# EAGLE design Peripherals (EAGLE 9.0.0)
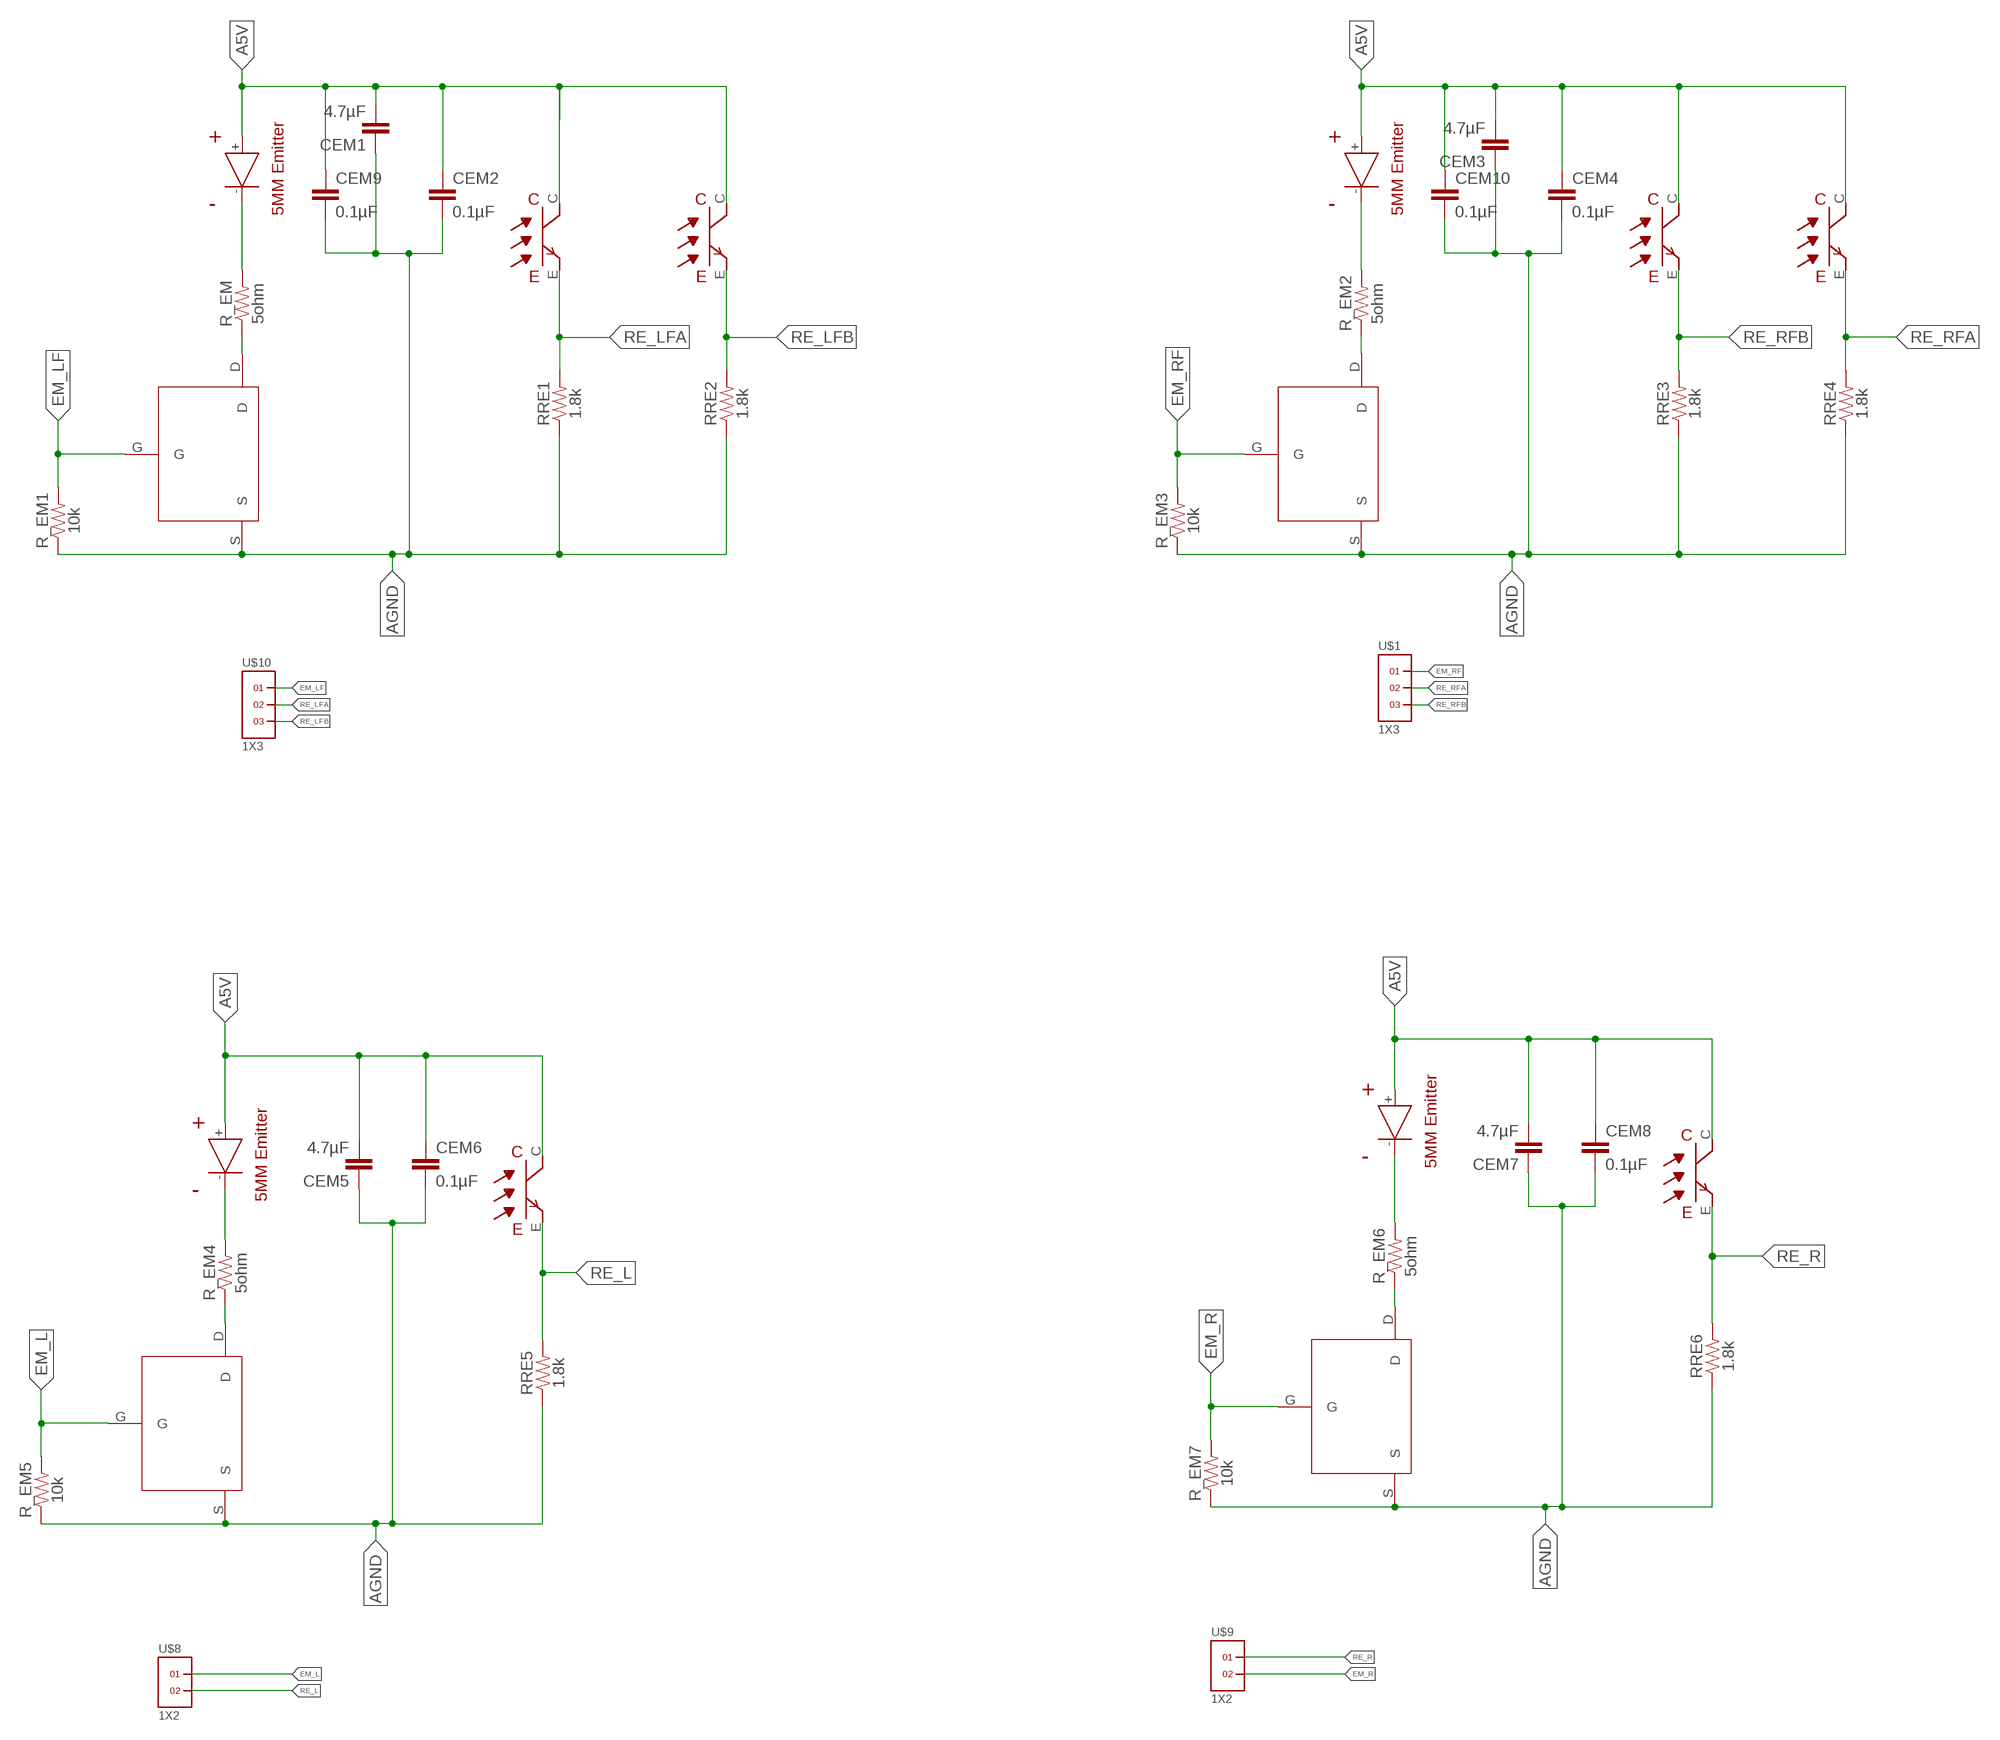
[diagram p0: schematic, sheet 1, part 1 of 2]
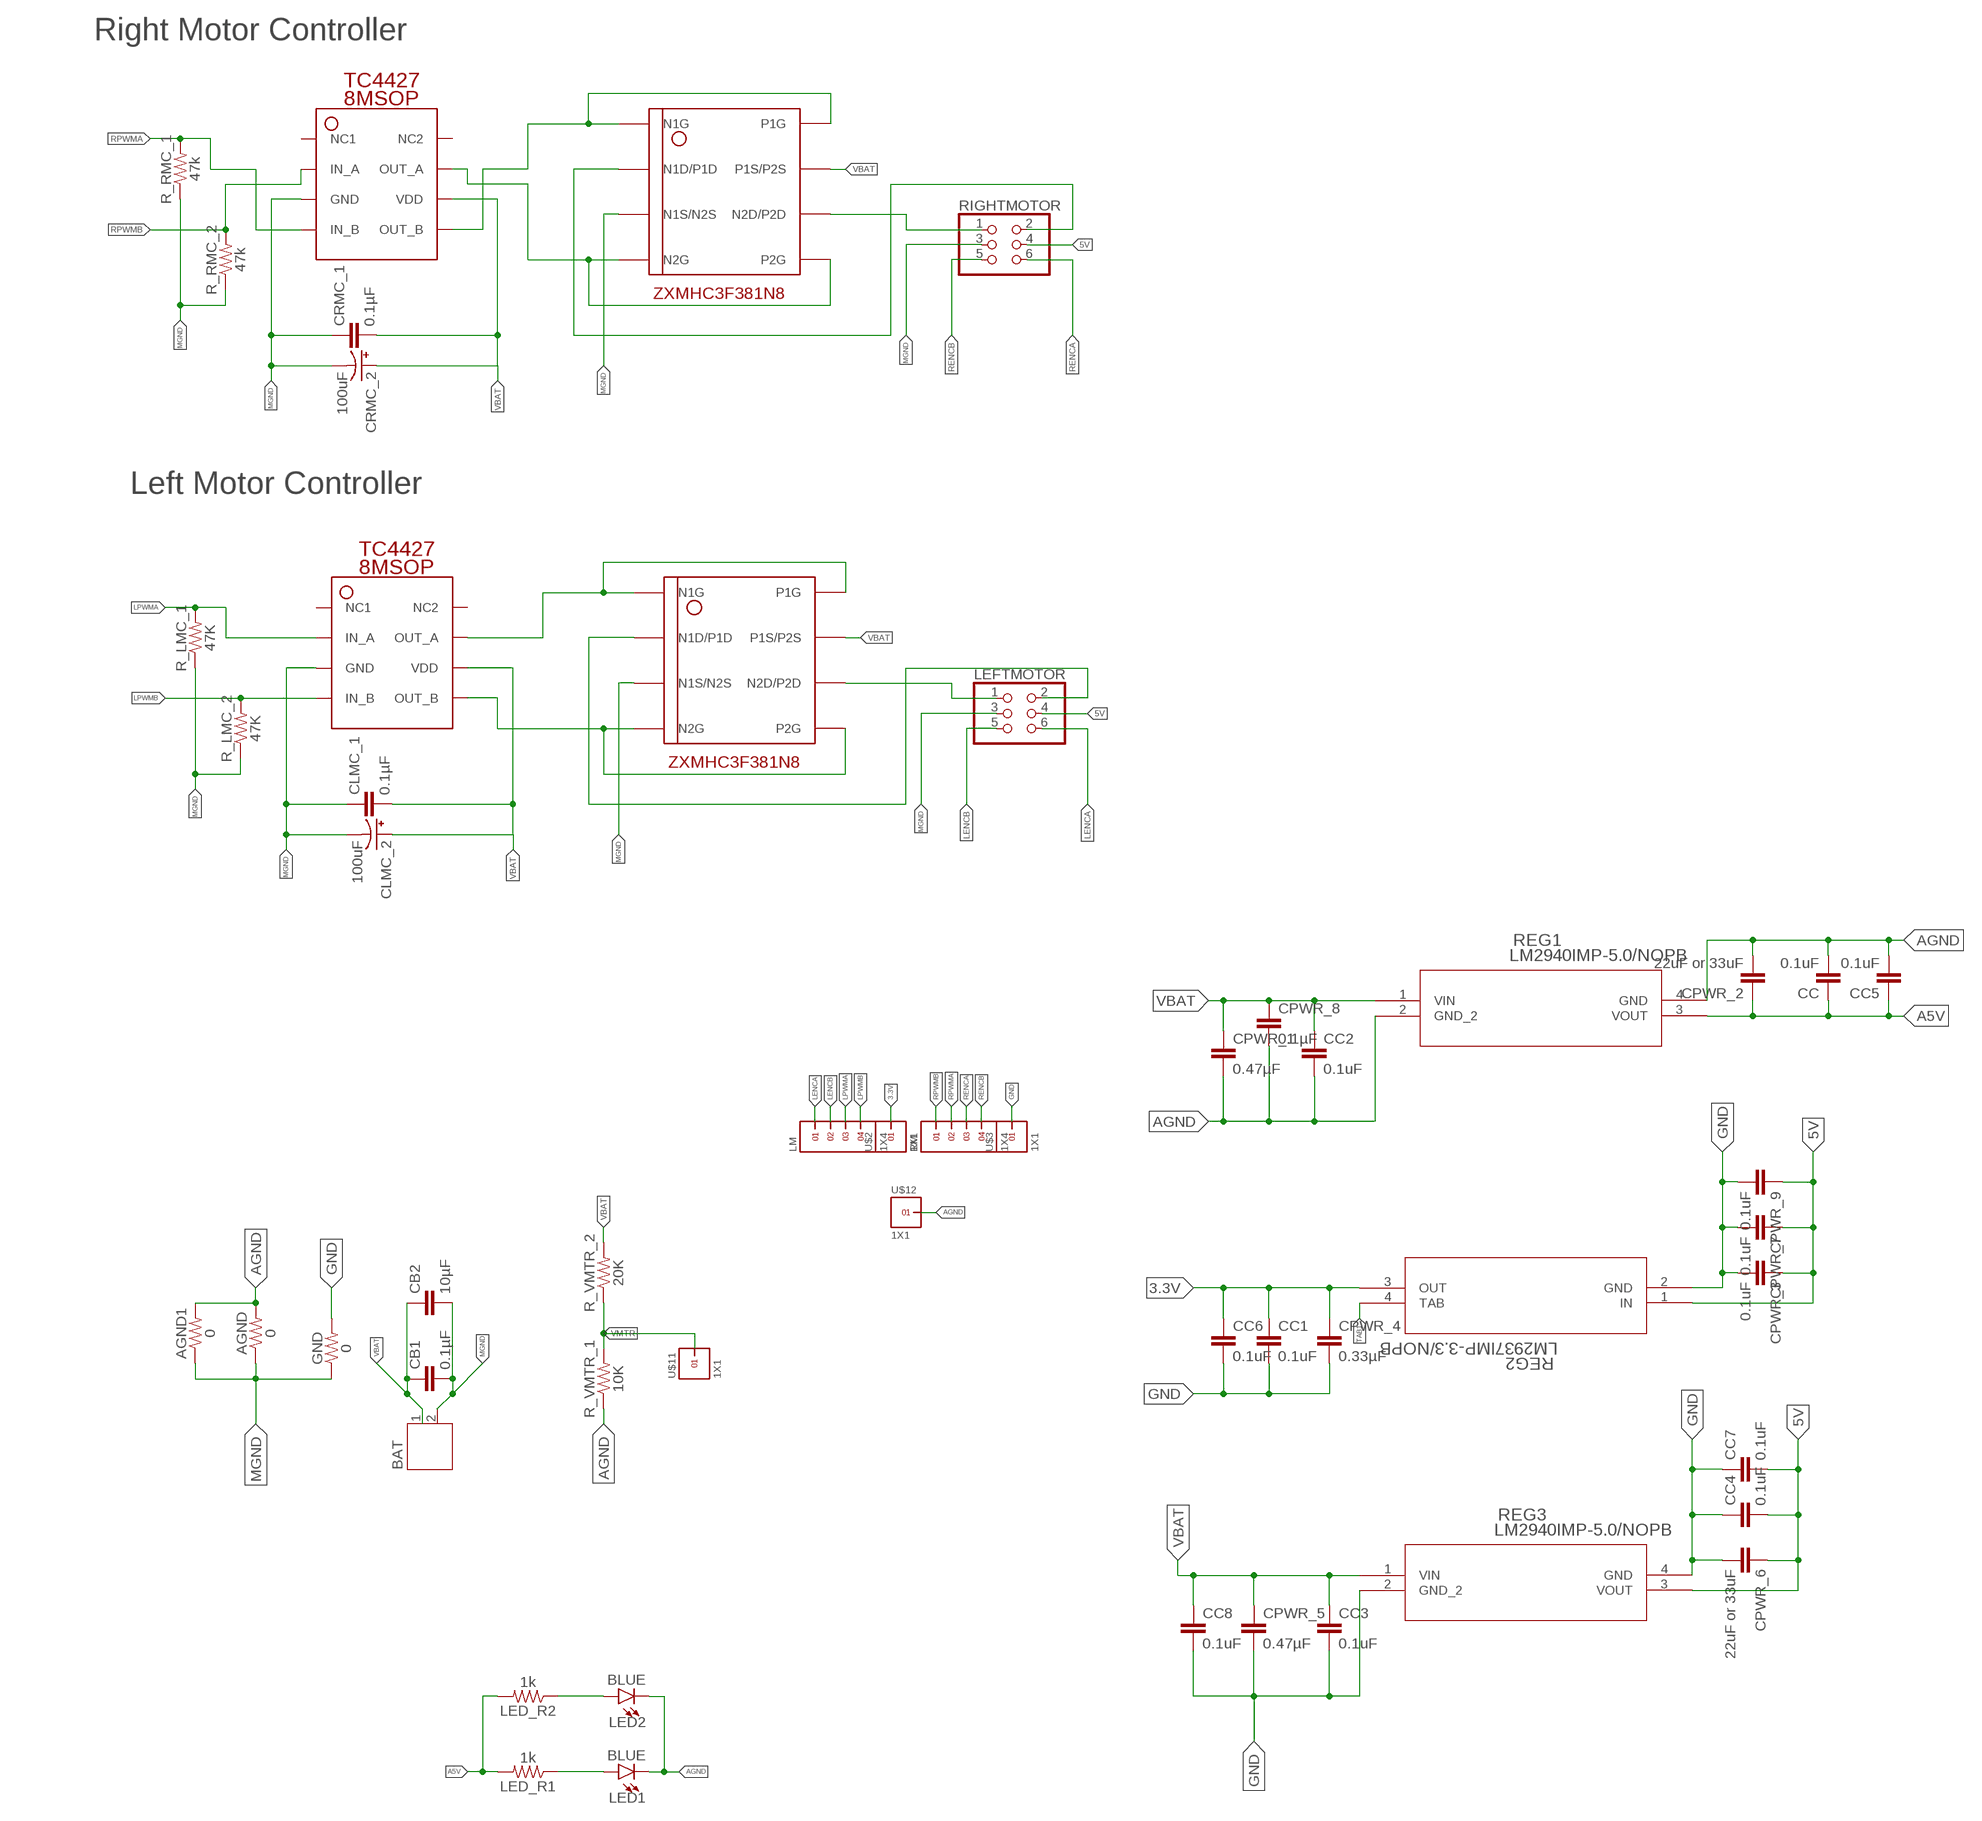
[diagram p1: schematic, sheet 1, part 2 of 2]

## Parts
AGND  0  0.75OHM-0805-1/4W-1%  [0805]
AGND1  0  0.75OHM-0805-1/4W-1%  [0805]
BAT  JST-PH2  [JST-PH2]
CB1  0.1µF  0.33UF/330NF-0805-50V-10%  [0805]
CB2  10µF  0.33UF/330NF-0805-50V-10%  [0805]
CC  0.1uF  0.33UF/330NF-0805-50V-10%  [0805]
CC1  0.1uF  0.33UF/330NF-0805-50V-10%  [0805]
CC2  0.1uF  0.33UF/330NF-0805-50V-10%  [0805]
CC3  0.1uF  0.33UF/330NF-0805-50V-10%  [0805]
CC4  0.1uF  0.33UF/330NF-0805-50V-10%  [0805]
CC5  0.1uF  0.33UF/330NF-0805-50V-10%  [0805]
CC6  0.1uF  0.33UF/330NF-0805-50V-10%  [0805]
CC7  0.1uF  0.33UF/330NF-0805-50V-10%  [0805]
CC8  0.1uF  0.33UF/330NF-0805-50V-10%  [0805]
CEM1  4.7µF  0.33UF/330NF-0805-50V-10%  [0805]
CEM2  0.1µF  0.33UF/330NF-0805-50V-10%  [0805]
CEM3  4.7µF  0.33UF/330NF-0805-50V-10%  [0805]
CEM4  0.1µF  0.33UF/330NF-0805-50V-10%  [0805]
CEM5  4.7µF  0.33UF/330NF-0805-50V-10%  [0805]
CEM6  0.1µF  0.33UF/330NF-0805-50V-10%  [0805]
CEM7  4.7µF  0.33UF/330NF-0805-50V-10%  [0805]
CEM8  0.1µF  0.33UF/330NF-0805-50V-10%  [0805]
CEM9  0.1µF  0.33UF/330NF-0805-50V-10%  [0805]
CEM10  0.1µF  0.33UF/330NF-0805-50V-10%  [0805]
CLMC_1  0.1µF  0.33UF/330NF-0805-50V-10%  [0805]
CLMC_2  100uF  100UF-POLAR-EIA7343-10V-10%(TANT)  [EIA7343]
CPWR_1  0.47µF  0.33UF/330NF-0805-50V-10%  [0805]
CPWR_2  22uF or 33uF  0.33UF/330NF-0805-50V-10%  [0805]
CPWR_3  0.1uF  0.33UF/330NF-0805-50V-10%  [0805]
CPWR_4  0.33µF  0.33UF/330NF-0805-50V-10%  [0805]
CPWR_5  0.47µF  0.33UF/330NF-0805-50V-10%  [0805]
CPWR_6  22uF or 33uF  0.33UF/330NF-0805-50V-10%  [0805]
CPWR_7  0.1uF  0.33UF/330NF-0805-50V-10%  [0805]
CPWR_8  0.1µF  0.33UF/330NF-0805-50V-10%  [0805]
CPWR_9  0.1uF  0.33UF/330NF-0805-50V-10%  [0805]
CRMC_1  0.1µF  0.33UF/330NF-0805-50V-10%  [0805]
CRMC_2  100uF  100UF-POLAR-EIA7343-10V-10%(TANT)  [EIA7343]
EM_L  EMITTER  [EMITTER]
EM_LF  EMITTER  [EMITTER]
EM_R  EMITTER  [EMITTER]
EM_RF  EMITTER  [EMITTER]
GND  0  0.75OHM-0805-1/4W-1%  [0805]
LED1  BLUE  LED-BLUE1206  [LED-1206]
LED2  BLUE  LED-BLUE1206  [LED-1206]
LED_R1  1k  0.75OHM-0805-1/4W-1%  [0805]
LED_R2  1k  0.75OHM-0805-1/4W-1%  [0805]
LEFTMOTOR  PINHD-2X3  [2X03]
LM  1X4  [1X4]
R_EM  5ohm  0.75OHM-0805-1/4W-1%  [0805]
R_EM1  10k  0.75OHM-0805-1/4W-1%  [0805]
R_EM2  5ohm  0.75OHM-0805-1/4W-1%  [0805]
R_EM3  10k  0.75OHM-0805-1/4W-1%  [0805]
R_EM4  5ohm  0.75OHM-0805-1/4W-1%  [0805]
R_EM5  10k  0.75OHM-0805-1/4W-1%  [0805]
R_EM6  5ohm  0.75OHM-0805-1/4W-1%  [0805]
R_EM7  10k  0.75OHM-0805-1/4W-1%  [0805]
R_LMC_1  47K  0.75OHM-0805-1/4W-1%  [0805]
R_LMC_2  47K  0.75OHM-0805-1/4W-1%  [0805]
R_RMC_1  47k  0.75OHM-0805-1/4W-1%  [0805]
R_RMC_2  47k  0.75OHM-0805-1/4W-1%  [0805]
R_VMTR_1  10K  0.75OHM-0805-1/4W-1%  [0805]
R_VMTR_2  20K  0.75OHM-0805-1/4W-1%  [0805]
RE_L  RECEIVER  [RECEIVER]
RE_LFA  RECEIVER  [RECEIVER]
RE_LFB  RECEIVER  [RECEIVER]
RE_R  RECEIVER  [RECEIVER]
RE_RFA  RECEIVER  [RECEIVER]
RE_RFB  RECEIVER  [RECEIVER]
REG1  LM2940IMP-5.0/NOPB  [MP04A]
REG2  LM2937IMP-3.3/NOPB  [MP04A]
REG3  LM2940IMP-5.0/NOPB  [MP04A]
RIGHTMOTOR  PINHD-2X3  [2X03]
RM  1X4  [1X4]
RRE1  1.8k  0.75OHM-0805-1/4W-1%  [0805]
RRE2  1.8k  0.75OHM-0805-1/4W-1%  [0805]
RRE3  1.8k  0.75OHM-0805-1/4W-1%  [0805]
RRE4  1.8k  0.75OHM-0805-1/4W-1%  [0805]
RRE5  1.8k  0.75OHM-0805-1/4W-1%  [0805]
RRE6  1.8k  0.75OHM-0805-1/4W-1%  [0805]
U$1  1X3  [1X3]
U$2  1X1  [1X1]
U$3  1X1  [1X1]
U$4  MCH3474  [MCH3474]
U$5  MCH3474  [MCH3474]
U$6  MCH3474  [MCH3474]
U$7  MCH3474  [MCH3474]
U$8  1X2  [1X2]
U$9  1X2  [1X2]
U$10  1X3  [1X3]
U$11  1X1  [1X1]
U$12  1X1  [1X1]
U$15  TC4427(8MSOP)  [TC4427(8MSOP)]
U$16  ZXMHC3F381N8  [ZXMHC3F381N8]
U$17  TC4427(8MSOP)  [TC4427(8MSOP)]
U$18  ZXMHC3F381N8  [ZXMHC3F381N8]

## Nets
3.3V: CC1.1 CC6.1 CPWR_4.1 REG2.3(OUT) U$2.1
5V: CC4.2 CC7.2 CPWR_3.1 CPWR_6.1 CPWR_7.1 CPWR_9.1 LEFTMOTOR.4 REG2.1(IN) REG3.3(VOUT) RIGHTMOTOR.4
A5V: CC5.1 CC.1 CEM1.2 CEM2.1 CEM3.2 CEM4.1 CEM5.2 CEM6.1 CEM7.2 CEM8.1 CEM9.1 CEM10.1 CPWR_2.1 EM_L.+ EM_LF.+ EM_R.+ EM_RF.+ LED_R1.2 LED_R2.2 RE_L.C RE_LFA.C RE_LFB.C RE_R.C RE_RFA.C RE_RFB.C REG1.3(VOUT)
AGND: AGND1.2 AGND.2 CC2.2 CC5.2 CC.2 CEM1.1 CEM2.2 CEM3.1 CEM4.2 CEM5.1 CEM6.2 CEM7.1 CEM8.2 CEM9.2 CEM10.2 CPWR_1.2 CPWR_2.2 CPWR_8.2 LED1.C LED2.C R_EM1.1 R_EM3.1 R_EM5.1 R_EM7.1 R_VMTR_1.1 REG1.2(GND_2) REG1.4(GND) RRE1.1 RRE2.1 RRE3.1 RRE4.1 RRE5.1 RRE6.1 U$4.S U$5.S U$6.S U$7.S U$12.1
EM_L: R_EM5.2 U$4.G U$8.1
EM_LF: R_EM1.2 U$5.G U$10.1
EM_R: R_EM7.2 U$7.G U$9.2
EM_RF: R_EM3.2 U$1.1 U$6.G
EMD_L: EM_L.- R_EM4.2
GND: CC1.2 CC3.2 CC4.1 CC6.2 CC7.1 CC8.2 CPWR_3.2 CPWR_4.2 CPWR_5.2 CPWR_6.2 CPWR_7.2 CPWR_9.2 GND.2 REG2.2(GND) REG3.2(GND_2) REG3.4(GND) U$3.1
L: LEFTMOTOR.2 U$16.N1D/P1D
LENCA: LEFTMOTOR.6 LM.1
LENCB: LEFTMOTOR.5 LM.2
LPWMA: LM.3 R_LMC_1.2 U$15.IN_A
LPWMB: LM.4 R_LMC_2.2 U$15.IN_B
MGND: AGND1.1 AGND.1 BAT.2 CB1.2 CB2.2 CLMC_1.1 CLMC_2.C(-) CRMC_1.1 CRMC_2.C(-) GND.1 LEFTMOTOR.3 R_LMC_1.1 R_LMC_2.1 R_RMC_1.1 R_RMC_2.1 RIGHTMOTOR.3 U$15.GND U$16.N1S/N2S U$17.GND U$18.N1S/N2S
N$1: R_EM.1 U$5.D
N$2: R_EM2.1 U$6.D
N$3: R_EM4.1 U$4.D
N$4: R_EM6.1 U$7.D
N$5: EM_LF.- R_EM.2
N$6: EM_RF.- R_EM2.2
N$7: EM_R.- R_EM6.2
N$8: LED1.A LED_R1.1
N$9: LEFTMOTOR.1 U$16.N2D/P2D
N$10: LED2.A LED_R2.1
N$36: RIGHTMOTOR.1 U$18.N2D/P2D
OUT_A: U$15.OUT_A U$16.N1G U$16.P1G
OUT_B: U$15.OUT_B U$16.N2G U$16.P2G
OUTA: U$17.OUT_B U$18.N1G U$18.P1G
OUTB: U$17.OUT_A U$18.N2G U$18.P2G
R: RIGHTMOTOR.2 U$18.N1D/P1D
RE_L: RE_L.E RRE5.2 U$8.2
RE_LFA: RE_LFA.E RRE1.2 U$10.2
RE_LFB: RE_LFB.E RRE2.2 U$10.3
RE_R: RE_R.E RRE6.2 U$9.1
RE_RFA: RE_RFB.E RRE4.2 U$1.2
RE_RFB: RE_RFA.E RRE3.2 U$1.3
RENCA: RIGHTMOTOR.6 RM.3
RENCB: RIGHTMOTOR.5 RM.4
RPWMA: R_RMC_1.2 RM.2 U$17.IN_B
RPWMB: R_RMC_2.2 RM.1 U$17.IN_A
TAB1: REG2.4(TAB)
VBAT: BAT.1 CB1.1 CB2.1 CC2.1 CC3.1 CC8.1 CLMC_1.2 CLMC_2.A(+) CPWR_1.1 CPWR_5.1 CPWR_8.1 CRMC_1.2 CRMC_2.A(+) R_VMTR_2.2 REG1.1(VIN) REG3.1(VIN) U$15.VDD U$16.P1S/P2S U$17.VDD U$18.P1S/P2S
VMTR: R_VMTR_1.2 R_VMTR_2.1 U$11.1
Unconnected: U$15.NC1 U$15.NC2 U$17.NC1 U$17.NC2

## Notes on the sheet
- Right Motor Controller
- Left Motor Controller

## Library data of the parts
AGND AGND1 GND LED_R1 LED_R2 R_EM R_EM1-R_EM7 R_LMC_1 R_LMC_2 R_RMC_1 R_RMC_2 R_VMTR_1 R_VMTR_2 RRE1-RRE6 = SparkFun-Resistors:0.75OHM: 0.75Ω resistor; PROD_ID: RES-08474; VALUE: 0.75
BAT = jst-ph:JST-PH2
CB1 CB2 CC CC1-CC8 CEM1-CEM10 CLMC_1 CPWR_1-CPWR_3 CPWR_5-CPWR_9 CRMC_1 = SparkFun-Capacitors:0.33UF/330NF: 0.33µF/330nF ceramic capacitors; PROD_ID: CAP-08469; VALUE: 0.33µF
CLMC_2 CRMC_2 = SparkFun-Capacitors:100UF-POLAR: 100µF polarized capacitors; PROD_ID: CAP-07890
CPWR_4 = SparkFun-Capacitors:0.33UF/330NF: 0.33µF/330nF ceramic capacitors; PROD_ID: CAP-08469
EM_L EM_LF EM_R EM_RF = sfh4550 & teft4300:EMITTER
LED1 LED2 = SparkFun-LED:LED-BLUE: Blue SMD LED; PROD_ID: DIO-09911
LEFTMOTOR RIGHTMOTOR = pinhead:PINHD-2X3: PIN HEADER
LM RM = headers(2mm):1X4
RE_L RE_LFA RE_LFB RE_R RE_RFA RE_RFB = sfh4550 & teft4300:RECEIVER
REG1 REG3 = LM2940IMP-5.0:LM2940IMP-5.0/NOPB; 3D_LIBRARY_NAME: National_LDO; BASE_PN: LM2940; COMP: TypeLDO; COPYRIGHT: Copyright C 2015 Accelerated Designs. All rights reserved; LIBRARY: ReferenceLM2940IMP; MANUFACTURER_PART_NUMBER: LM2940IMP5.0NOPB; PIN: Count4; SYMBOL: NameLM2940IMP50; TYPE: LM2940IMP5.0; VENDOR: National Semiconductor; VERSION: 1
REG2 = LM2937IMP-3.3:LM2937IMP-3.3/NOPB; COPYRIGHT: Copyright C 2015 Accelerated Designs. All rights reserved; MANUFACTURER_PART_NUMBER: lm2937imp3_3nopb; VENDOR: National Semiconductor
U$1 U$10 = headers(2mm):1X3
U$2 U$3 U$11 U$12 = headers(2mm):1X1
U$4-U$7 = MCH3474:MCH3474
U$8 U$9 = headers(2mm):1X2
U$15 U$17 = TC4427(8MSOP):TC4427(8MSOP)
U$16 U$18 = ZXMHC3F381N8:ZXMHC3F381N8

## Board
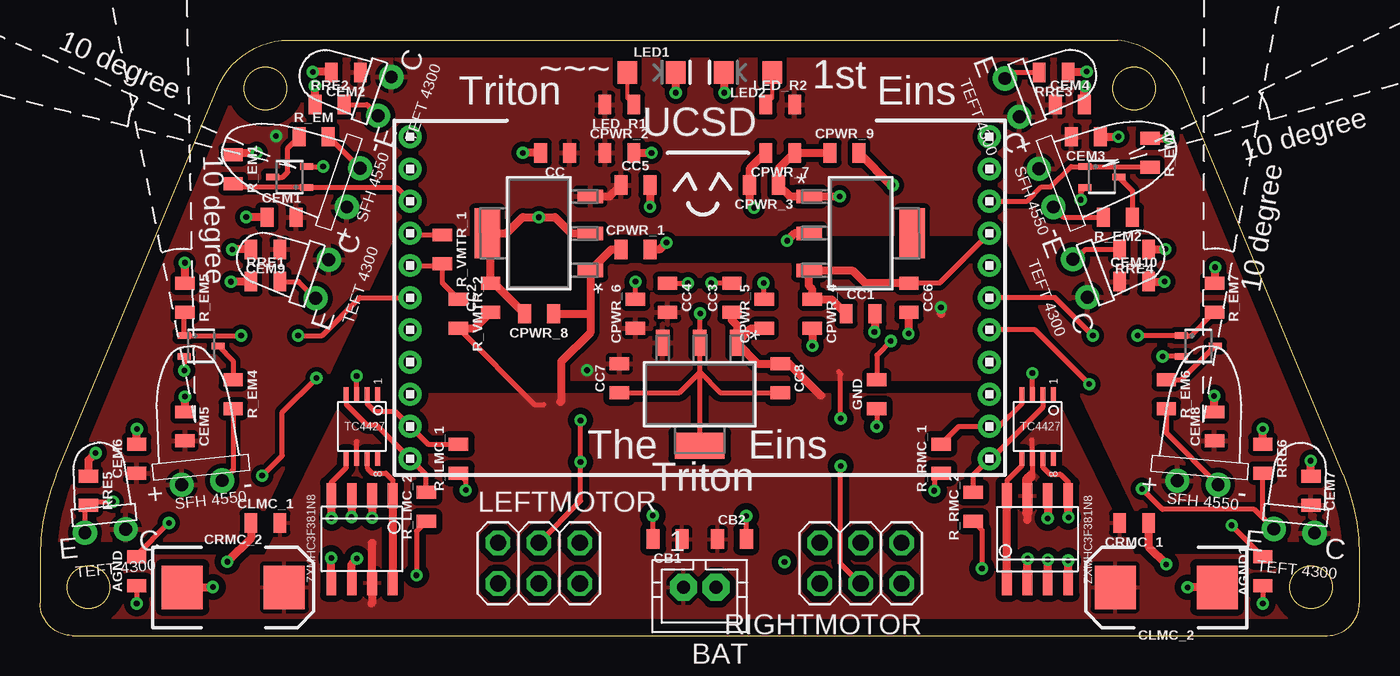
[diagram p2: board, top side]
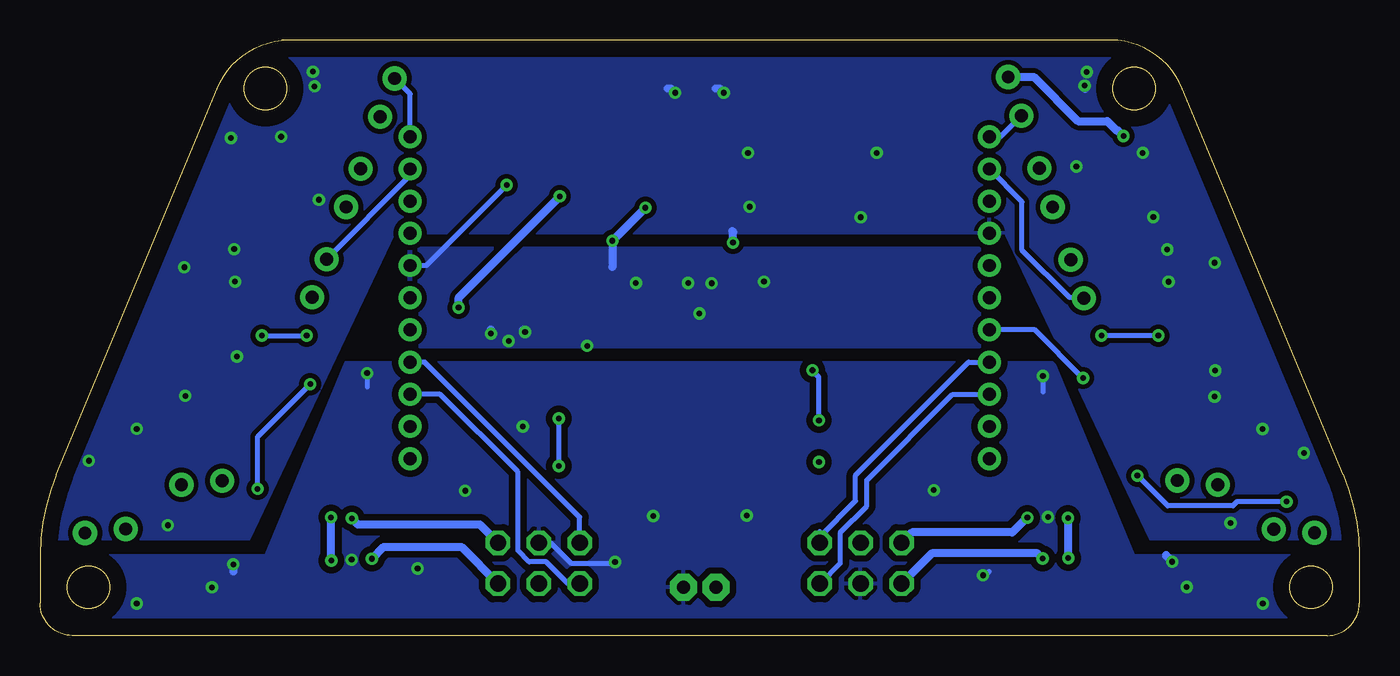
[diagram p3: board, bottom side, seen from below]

Size 82 x 37 mm. Coordinates in mm from the lower left corner, seen from the top.
Outline: 2,0 80,0 arc90 82,2 82,5 arc23 81,10 71,34 arc61 67,37 15,37 arc61 11,34 1,10 arc23 0,5 0,2 arc90 2,0
Outline: circle at 14,34 radius 1.3
Outline: circle at 68,34 radius 1.3
Outline: circle at 3,3 radius 1.3
Outline: circle at 79,3 radius 1.3
Copper layers (1*16): Top 0.035mm / dielectric 1.5mm / Bottom 0.035mm
Design rules "default": minimum track width 6mil, minimum drill 0.35mm, track to track 6mil, track to pad 6mil, pad to pad 6mil, via to via 6mil, smd to smd 6mil, copper to edge 40mil, drill to drill 6mil, minimum pad ring 10mil, minimum via ring 8mil, stop-mask expansion 4mil, vias tented up to drill 0mil, thermal gap 10mil

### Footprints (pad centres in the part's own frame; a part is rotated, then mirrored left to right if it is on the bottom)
0805 = smd 0.8 x 1.2: 1 -0.9,0; 2 0.9,0
JST-PH2 = drill 0.813 pad 1.676 octagon: 1 1,0; 2 -1,0
EIA7343 = smd 2.55 x 2.7: A 3.17,0; C -3.17,0
EMITTER = drill 0.8 pad 1.5: + -1.27,-0.5; - 1.27,-0.5
LED-1206 = smd 1.2 x 1.4: A -1.5,0; C 1.5,0
2X03 = drill 1.016 octagon: 1 -2.54,-1.27; 2 -2.54,1.27; 3 0,-1.27; 4 0,1.27; 5 2.54,-1.27; 6 2.54,1.27
1X4 = drill 0.8 pad 1.422: 1 -3,0; 2 -1,0; 3 1,0; 4 3,0
RECEIVER = drill 0.8 pad 1.5: C 1.27,-0.5; E -1.27,-0.5
MP04A = smd 1.6 x 0.838: 1 -3.2,2.3; 2 -3.2,0; 3 -3.2,-2.3 | smd 1.6 x 3.099: 4 3.2,0
1X3 = drill 0.8 pad 1.422: 1 -2,0; 2 0,0; 3 2,0
1X1 = drill 0.8 pad 1.422: 1 0,0
MCH3474 = smd 0.406 x 0.813: D 0,1.05; G -0.65,-1.05; S 0.65,-1.05
1X2 = drill 0.8 pad 1.422: 1 -1,0; 2 1,0
TC4427(8MSOP) = smd 0.95 x 0.3: GND -1.975,-0.325; IN_A -1.975,0.325; IN_B -1.975,-0.975; NC1 -1.975,0.975; NC2 1.975,0.975; OUT_A 1.975,0.325; OUT_B 1.975,-0.975; VDD 1.975,-0.325
ZXMHC3F381N8 = smd 0.6 x 1.55: N1D/P1D -0.635,-2.7; N1G -1.905,-2.7; N1S/N2S 0.635,-2.7; N2D/P2D 0.635,2.7; N2G 1.905,-2.7; P1G -1.905,2.7; P1S/P2S -0.635,2.7; P2G 1.905,2.7

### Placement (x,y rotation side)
AGND  6,4 90 top
AGND1  76,4 90 top
BAT  41,3 180 top
CB1  39,6 180 top
CB2  43,6 0 top
CC  32,30 180 top
CC1  51,20 0 top
CC2  28,21 90 top
CC3  43,21 90 top
CC4  39,21 270 top
CC5  37,28 0 top
CC6  54,21 270 top
CC7  36,16 90 top
CC8  46,16 270 top
CEM1  15,26 0 top
CEM2  19,35 180 top
CEM3  65,31 180 top
CEM4  64,33 0 top
CEM5  9,13 270 top
CEM6  6,11 90 top
CEM7  79,9 270 top
CEM8  73,13 90 top
CEM9  14,24 180 top
CEM10  68,22 0 top
CLMC_1  14,7 0 top
CLMC_2  70,3 180 top
CPWR_1  37,24 0 top
CPWR_2  36,30 0 top
CPWR_3  45,28 180 top
CPWR_4  48,20 270 top
CPWR_5  45,20 90 top
CPWR_6  37,20 90 top
CPWR_7  46,30 180 top
CPWR_8  31,20 180 top
CPWR_9  50,30 0 top
CRMC_1  68,7 180 top
CRMC_2  12,3 0 top
EM_L  10,10 6.2 top
EM_LF  19,28 71.1 top
EM_R  72,10 354.8 top
EM_RF  63,28 290.7 top
GND  52,15 90 top
LED1  38,35 0 top
LED2  44,35 180 top
LED_R1  36,33 180 top
LED_R2  46,33 0 top
LEFTMOTOR  31,4.5 0 top
LM  23,14 270 top
R_EM  17,31 0 top
R_EM1  12,28.99 270 top
R_EM2  67,26 180 top
R_EM3  69,30 270 top
R_EM4  12,15 270 top
R_EM5  9,21 270 top
R_EM6  70,15 270 top
R_EM7  73,21 270 top
R_LMC_1  26,11 90 top
R_LMC_2  24,8 90 top
R_RMC_1  56,11 90 top
R_RMC_2  58,8 90 top
R_VMTR_1  25,24 270 top
R_VMTR_2  26,20 270 top
RE_L  4,7 5.4 top
RE_LFA  17.06,22.32 71.1 top
RE_LFB  20.94,33.68 71.1 top
RE_R  78,7 354.3 top
RE_RFA  60.88,33.61 290.7 top
RE_RFB  65.12,22.39 290.7 top
REG1  31,25 180 top
REG2  51,25 0 top
REG3  41,15 270 top
RIGHTMOTOR  51,4.5 180 top
RM  59,14 90 top
RRE1  14,22 0 top
RRE2  18,33 0 top
RRE3  63,35 180 top
RRE4  68,24 180 top
RRE5  3,9 270 top
RRE6  76,11 270 top
U$1  59,29 90 top
U$2  59,25 0 top
U$3  59,23 0 top
U$4  10,18 270 top
U$5  15.5,28.5 90 top
U$6  66,28.5 270 top
U$7  72,18 270 top
U$8  23,20 270 top
U$9  59,20 90 top
U$10  23,29 90 top
U$11  23,23 0 top
U$12  23,25 0 top
U$15  20,13 270 top
U$16  20,6 180 top
U$17  62,13 270 top
U$18  62,6 0 top

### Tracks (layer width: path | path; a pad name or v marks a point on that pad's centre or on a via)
3.3V
  Top 0.305: U$2.1 55.9,21.9 CC6.1
  Top 0.508: REG2.3 47.79,21.72 48,21.51 CPWR_4.1 49.2,20.9 CC1.1 | REG2.3 | CC6.1 51.29,21.9 50.53,22.66 47.82,22.66 REG2.3
5V  (via drill 0.35)
  Top 0.305: LEFTMOTOR.4 33.6,8.37 v33.6,10.78 v33.59,10.79 v33.59,13.38 | RIGHTMOTOR.4 49.75,4.48 v49.75,10.53 v49.76,10.54 | v49.76,13.49 49.76,16.27 49.63,16.4
  Top 0.508: v49.7,27.3 REG2.1 46.6,27.3 CPWR_3.1 45.9,29 CPWR_7.1 CPWR_9.1 | v55.99,20.39 55.99,20.01 56,20
  Bottom 0.305: v49.76,10.54 v49.76,13.49 | v33.59,13.38 33.59,16.07 33.99,16.47 v33.99,16.49
  Bottom 0.508: v55.99,20.39 55.99,21.01 v49.7,27.3
  pour Top (isolate 0.305): 19,16 63,16 60,23 22,23
A5V  (via drill 0.35)
  Top 0.508: REG1.3 35.4,27.3 CC5.1
  Bottom 0.508: RE_LFB.C 20.24,34.72 17.49,31.97 15.66,31.97 15.08,31.39 15,31.39 v14.66,31.05
  pour Top (isolate 0.305): -4,6 13,6 22,25 60,25 69,6 84,6 70,38 11,38
AGND  (via drill 0.35)
  Top 0.305: AGND.2 6,5 v8,7 | AGND1.2 74.07,6.83 v74.07,6.86 | U$4.S 8.95,16.63 v8.96,16.48 | U$5.S v17.59,29.15 | U$7.S v69.77,17.35 | U$6.S 64.68,27.58 v64.68,27.09 | U$12.1 23.1,24.9 R_VMTR_1.1
  Top 0.508: CC.2 v30,30 | CPWR_2.2 v38,30 | RRE5.1 3,10.91 v3.44,11.35 | CEM6.2 v6,12.83 v6.01,12.84 | CEM5.1 v9,14.85 | R_EM5.1 9,22.75 v8.99,23.17 | RRE1.1 12.23,22 v11.86,21.99 | CEM9.2 v11.94,24 | CEM1.1 13.25,26 v12.8,26.01 | R_EM1.1 12.11,30 v13.46,30 | RRE2.1 17.1,34.01 v17.08,34.18 | CEM2.2 18.07,35.03 v16.94,35.03 16.85,34.94 | RRE3.1 63.95,35.05 v65.05,35.05 | 64.94,33.04 CEM4.2 64.9,34.08 v64.95,34.13 | CEM3.1 v67.02,31 | RRE4.1 68.92,24.02 v69.94,24.02 | CEM10.2 v69.89,22 | R_EM7.1 73.04,21.94 v73.04,22.89 | CEM8.2 72.98,13.92 v72.98,14.9 | RRE6.1 v76,12.85 | CEM7.1 78.98,9.92 v78.98,10.87 | REG1.4 28,25 | 28,25 29,25 30,26 v31,26 32,26 33,25 REG1.2 | CPWR_1.2 37.92,24.02 | CPWR_8.2 28.2,21.9 CC2.2 28,25 | CC5.2 v37.9,26.65 | 37.92,24.02 37.96,23.98 | 37.92,24.02 38.53,24.02 v38.93,24.42 | LED1.C v39.5,33.75 v39.51,33.74 | LED2.C 42.5,33.77 v42.53,33.74 | R_EM3.1 70.12,30.9 v70.14,30.92
  Bottom 0.305: v74.07,6.86 74.07,6.93 74,7 | 9.02,22.98 9,23
  Bottom 0.508: v38.93,24.42 38.93,25.07 38.99,25.13 | v39.51,33.74 39.77,34 40,34 | v42.53,33.74 42.79,34 43,34 | v17.08,34.18 17.09,34 17,34 | v64.95,34.13 65,34.08 65,34 | v70.14,30.92 70.06,31 70,31
  pour Bottom (isolate 0.305): -4,6 13,6 22,25 60,25 69,6 84,6 82,10 70,38 12,38
EM_L  (via drill 0.35)
  Top 0.305: R_EM5.2 8.95,20.05 U$4.G v12.49,18.65 | v16.03,18.65 17.52,18.65 19.87,21 U$8.1
  Bottom 0.305: v12.49,18.65 v16.03,18.65
EM_LF
  Top 0.305: R_EM1.2 12.24,27.85 U$5.G 22.15,27.85 U$10.1
EM_R  (via drill 0.35)
  Top 0.305: R_EM7.2 71.55,18.65 U$7.G v68.22,18.65 | v65.44,18.65 63.09,21 U$9.2
  Bottom 0.305: v68.22,18.65 v65.44,18.65
EM_RF
  Top 0.305: R_EM3.2 68.95,29.15 U$6.G 64.08,29.15 62.81,27.88 62.24,27.88 61.36,27 U$1.1
EMD_L
  Top 0.305: R_EM4.2 12,10.32 EM_L.-
GND  (via drill 0.35)
  Top 0.305: REG3.4 41,16.37 | 41,16.37 REG3.2 41,20 v41.02,20.02 | CC7.1 39.73,15.1 41,16.37 | 41,16.37 42.27,15.1 CC8.2 | CPWR_6.2 v37,21.99 v37.01,22 | CC4.1 v40.26,21.9 | CC3.2 v41.72,21.91 | CPWR_5.2 45,21.88 v44.97,21.91 | v52.88,18.31 52,17.43 GND.2
  Top 0.508: CPWR_4.2 v48,18.01 | CC1.2 51.9,18.91 v51.86,18.87 | CC6.2 53.98,20.08 v53.98,18.77 | v44.38,26.59 44.1,26.87 CPWR_3.2 44.1,29 CPWR_7.2 | REG2.2 46.89,25 v46.43,24.54 | CPWR_9.2 52.9,28 v53,28
  Bottom 0.305: v53,28 58,23 U$3.1
  Bottom 0.508: v48,18.01 v48,18 | v51.86,18.87 51.99,19 52,19 | v53.98,18.77 53.98,19.02 54,19 | v44.38,26.59 v46.43,24.54 46.43,22.9
  pour Bottom (isolate 0.305): 20,18 23,24 59,24 62,18
L  (via drill 0.35)
  Top 0.508: U$16.N1D/P1D 20.63,7.48 v20.63,7.33
  Bottom 0.508: v20.63,7.33 20.62,7.37 21.57,6.42 27.81,6.42 LEFTMOTOR.2
LENCA
  Bottom 0.305: 33.54,6.46 LEFTMOTOR.6 33.54,6.14 31.31,8.37 31.31,9.98 24.29,17 LM.1
LENCB
  Bottom 0.305: LEFTMOTOR.5 32.28,4.49 32.28,6.39 30.62,8.05 30.62,9.67 25.29,15 LM.2
LPWMA
  Top 0.305: U$15.IN_A 20.33,14.4 20.79,13.93 22.07,13.93 LM.3 24.1,11.9 R_LMC_1.2
LPWMB
  Top 0.305: R_LMC_2.2 24,10 LM.4 20.89,13.11 20.28,13.11 19.02,14.37 U$15.IN_B
  Bottom 0.305: 22.95,11 LM.4
MGND  (via drill 0.35)
  Top 0.305: CB1.2 38.1,7.45 v38.08,7.47 | CB2.2 v43.9,7.42 v43.89,7.43 | R_RMC_2.1 58.54,6.56 v58.54,4.17 | R_LMC_2.1 23.39,6.49 v23.39,3.75 | GND.1 v52,13 | AGND.1 v6,2 | AGND1.1 v76,2 | U$15.GND 19.67,15.9 v19.67,16.13 | U$17.GND 61.67,15.92 v61.68,16.31 | R_RMC_1.1 55.58,9.68 v55.58,9 | R_LMC_1.1 26.45,9.65 v26.45,9.04
  Top 0.508: U$16.N1S/N2S 19.37,7.38 v19.35,7.37 | CRMC_2.C 10.71,3 v10.73,3.02 | U$18.N1S/N2S v62.64,4.72 | CLMC_2.C v71.33,3 | CLMC_1.1 13.1,6.06 v11.63,4.59 | CRMC_1.1 68.9,5.53 v70,4.43
  Bottom 0.305: RIGHTMOTOR.3 50.27,5.77 49,4.5 46.35,4.5 v46.27,4.58 | v23.39,3.75 23.25,3.75 23,4 | v19.67,16.13 19.66,15.89 19.66,15.13 | v61.68,16.31 61.67,15.92 61.67,15.44
  Bottom 0.508: v11.63,4.59 12,4.96 12,5 | v70,4.43 70,4
  pour Bottom (isolate 0.406): -4,-1 -3,5 14,5 19,17 63,17 68,5 84,5 84,-1
N$1
  Top 0.305: U$5.D 15.08,28.5 15.39,28.81 15.39,30.29 R_EM.1
N$2
  Top 0.305: U$6.D 67.9,27.65 R_EM2.1
N$3
  Top 0.305: U$4.D 12,17.05 R_EM4.1
N$4
  Top 0.305: R_EM6.1 70.95,15.9 U$7.D
N$5
  Top 0.305: R_EM.2 17.92,31 EM_LF.-
N$6
  Top 0.305: EM_RF.- 63.62,26 R_EM2.2
N$7
  Top 0.305: R_EM6.2 70,12.61 EM_R.-
N$8
  Top 0.254: LED_R1.1 36.5,33.4 LED1.A
N$9  (via drill 0.35)
  Top 0.508: U$16.N2D/P2D 19.37,4.47 v19.69,4.79
  Bottom 0.508: v19.69,4.79 20.01,5.11 26.58,5.11 LEFTMOTOR.1
N$10
  Top 0.254: LED2.A 45.5,33.4 LED_R2.1
N$36  (via drill 0.35)
  Top 0.508: U$18.N2D/P2D 62.64,7.45 v62.63,7.29
  Bottom 0.508: RIGHTMOTOR.1 54.67,6.9 62.24,6.9 v62.63,7.29
OUT_A
  Top 0.305: 20.33,10.58 U$15.OUT_A 20.33,10.41 20.63,10.1 21.48,10.1 21.91,9.67 21.91,9.66 U$16.N1G
  Top 0.508: U$16.N1G U$16.P1G
OUT_B  (via drill 0.35)
  Top 0.305: U$16.N2G 18.09,9.51 19.02,10.44 U$15.OUT_B
  Top 0.508: U$16.P2G v18.09,4.81 v18.09,4.82 | v18.11,7.31 18.11,8.69 U$16.N2G
  Bottom 0.508: v18.09,4.82 18.09,7.29 v18.11,7.31
OUTA
  Top 0.305: U$17.OUT_B 61.03,10.56 60.09,9.63 U$18.P1G
  Top 0.508: U$18.N1G U$18.P1G
OUTB  (via drill 0.35)
  Top 0.305: 62.33,10.55 U$17.OUT_A 62.33,10.47 62.75,10.04 63.41,10.04 63.91,9.55 U$18.P2G
  Top 0.508: U$18.N2G v63.91,4.66 v63.9,4.67 | v63.92,7.35 63.92,8.69 U$18.P2G
  Bottom 0.508: v63.9,4.67 63.9,7.33 v63.92,7.35
R  (via drill 0.35)
  Top 0.508: U$18.N1D/P1D 61.36,4.77 v61.38,4.78
  Bottom 0.508: v61.38,4.78 60.65,5.51 55.82,5.51 RIGHTMOTOR.2
RE_L  (via drill 0.35)
  Top 0.305: RE_L.E 2.78,7.88 RRE5.2 3.23,8.33 v4.52,8.33 | v13.8,9.94 15.05,11.19 15.05,13.89 v17.17,16.01
  Bottom 0.305: v4.52,8.33 7.6,8.33 7.86,8.07 11.91,8.07 13.78,9.94 v13.8,9.94 | v17.17,16.01 20.16,19 U$8.2
RE_LFA
  Top 0.305: RRE1.2 16.08,22 RE_LFA.E
  Bottom 0.305: RE_LFA.E 17.16,21 18,21 20.96,23.96 20.96,26.96 U$10.2
RE_LFB
  Top 0.305: RRE2.2 20.32,33 RE_LFB.E
  Bottom 0.305: RE_LFB.E 22.32,31 U$10.3
RE_R  (via drill 0.35)
  Top 0.305: RRE6.2 76,7.31 RE_R.E 75.47,7.85 69.76,7.85 v68.49,9.12 | U$9.1 61.84,19 v65.21,15.63
  Bottom 0.305: v68.49,9.12 68.49,12.35 v65.21,15.63
RE_RFA
  Top 0.305: RE_RFB.E 64.4,23.4 65,24 RRE4.2
  Bottom 0.305: RE_RFB.E 59,28.6 U$1.2
RE_RFB
  Top 0.305: RE_RFA.E 60.34,35 RRE3.2
  Bottom 0.305: U$1.3 59,33.66 RE_RFA.E
RENCA
  Bottom 0.305: 51.59,4.59 51.6,4.6 | 51.6,4.6 52.3,5.3 52.3,10.17 57.13,15 RM.3 | RIGHTMOTOR.6 49.19,3.23 50.56,4.6 51.6,4.6
RENCB
  Bottom 0.305: RIGHTMOTOR.5 48.46,7.36 58.1,17 RM.4
RPWMA
  Top 0.305: U$17.IN_B 61.03,14.38 59.64,13 RM.2 57.1,13 R_RMC_1.2
RPWMB
  Top 0.305: R_RMC_2.2 58,10 RM.1 59.13,11 62.33,14.2 U$17.IN_A
VBAT
  Top 0.305: U$15.VDD 19.67,12.05 19.66,12.07 | 61.64,12.17 61.67,12.13 U$17.VDD 61.67,10.02 61.57,9.91 | R_VMTR_2.2 30.74,14.36 31.31,14.36
  Top 0.508: CC3.1 43,19.6 43.3,19.3 REG3.1 | REG3.1 44.2,19.1 CPWR_5.1 | REG3.1 44.6,16.9 CC8.1 46.56,16.9 48.54,14.92 | 34.2,20 REG1.1 35.5,24 CPWR_1.1 | 34.2,20 34.2,18.83 32.39,17.02 32.39,14.58 32.34,14.53 | CPWR_8.1 34.2,20 | R_VMTR_2.2 27,19.1 CC2.1 | 20.61,5.77 20.63,5.74 U$16.P1S/P2S 20.63,2.05 20.6,2.01 | 61.36,7.63 61.36,7.18
  Top 0.61: U$18.P1S/P2S 61.36,7.63 | U$18.P1S/P2S 61.36,9.7 61.57,9.91
  pour Top (isolate 0.406): -4,0 -3.98,4.94 14,5 19,15 63,15 68,5 84,5 84,-1 -4,-1
VMTR
  Top 0.305: R_VMTR_2.1 25,21.9 25,23.02 | 25,23.02 R_VMTR_1.2 | U$11.1 24.98,23 25,23.02

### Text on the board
tNames: ~~~ | 1st | Triton | UCSD | Eins | The | Eins | Triton

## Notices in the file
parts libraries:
SparkFun-Capacitors: Licensing: Creative Commons ShareAlike 4.0 International - https://creativecommons.org/licenses/by-sa/4.0
